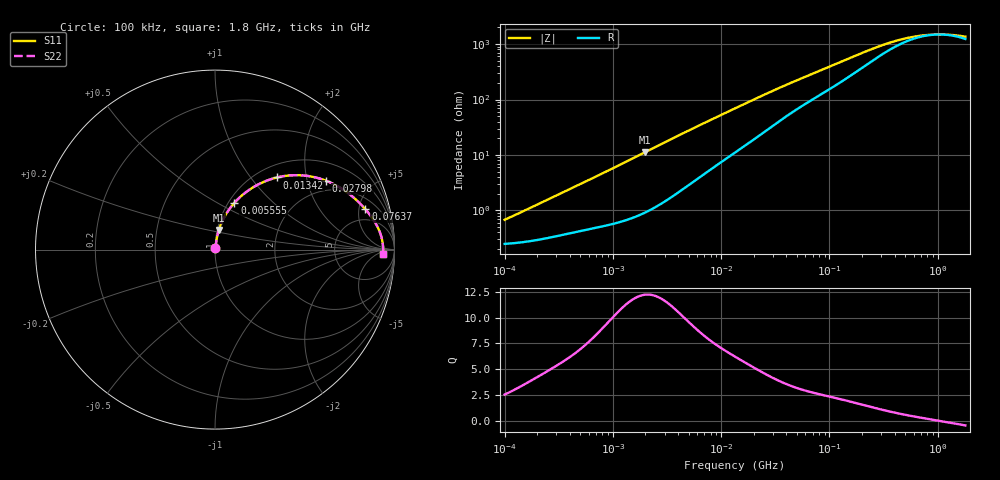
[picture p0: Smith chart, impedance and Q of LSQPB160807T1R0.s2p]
! LSQPB160807T1R0  S-PARAMETER MODEL  ( General Type )
! Model Generated by TAIYO YUDEN Corporation (http://www.ty-top.com)
! Version 1.0
! TAIYO YUDEN Control No. 110308NG25SB-FKC
! Copyright(c) 2011 TAIYO YUDEN CO.,LTD. All Rights Reserved.
! Product Description (link to TY-COMPAS)
! https://ds.yuden.co.jp/TYCOMPAS/or/detail?pn=LSQPB160807T1R0M&u=M
! Products Name : Inductors
! Characteristics :
!  Inductance : 1.0 uH , SRF(min) : 700 MHz , DC Resistance(max) : 0.299 Ohm
!  Rated Current : Saturation :510 mA , Temp Rise : 650 mA (40 degC)
!  Case Size : 1.6 x 0.8 / 0.063 x 0.031 [mm/inch] , Thickness : 0.7 / 0.028 [mm/inch]
!  (Conditions: Temperature = 25 degC , DC Bias Current/Voltage = 0A / 0V)
! External Node Assignments :
!  1  o---GGG---o  2
! GND o---------o GND
! Frequency Range : 0.1MHz  -  1800MHz  [ 402 STEP ]
# MHz S RI R 50
! Freq[MHz].  S11 Real  S11 Imag  S21 Real  S21 Imag  S12 Real  S12 Imag  S22 Real  S22 Imag
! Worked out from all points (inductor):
!   401 points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, 100 kHz to 1.8 GHz, reference 50 ohm
!   read as one part in series: L = 994 nH near 124.7 kHz
!   highest Q = 12.2 at 1.985 MHz (marker M1), where L = 898 nH
!   self-resonance near 1.02 GHz
!   S11 on the Smith chart (normalised r, x): 100 kHz: 1.00, +0.01; 5.555 MHz: 1.07, +0.60; 13.42 MHz: 1.22, +1.37; 27.98 MHz: 1.61, +2.63; 76.37 MHz: 3.23, +5.86; 1.8 GHz: 26, -11
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0.1  0.00252 0.00627  0.9975 -0.00627  0.9975 -0.00627  0.00252 0.00627
0.137498  0.0027 0.00856  0.9973 -0.00856  0.9973 -0.00856  0.0027 0.00856
0.516129  0.00519 0.0301  0.9948 -0.0301  0.9948 -0.0301  0.00519 0.0301
1.076226  0.00958 0.0606  0.9904 -0.0606  0.9904 -0.0606  0.00958 0.0606
1.985446  0.0211 0.1086  0.9789 -0.1086  0.9789 -0.1086  0.0211 0.1086
2.66389  0.0333 0.1425  0.9667 -0.1425  0.9667 -0.1425  0.0333 0.1425
3.942096  0.063 0.2004  0.937 -0.2004  0.937 -0.2004  0.063 0.2004
5.554714  0.1084 0.261  0.8916 -0.261  0.8916 -0.261  0.1084 0.261
8.632747  0.2044 0.3421  0.7956 -0.3421  0.7956 -0.3421  0.2044 0.3421
13.41641  0.3467 0.4023  0.6533 -0.4023  0.6533 -0.4023  0.3467 0.4023
19.37354  0.4872 0.4135  0.5128 -0.4135  0.5128 -0.4135  0.4872 0.4135
27.97575  0.6201 0.3832  0.3799 -0.3832  0.3799 -0.3832  0.6201 0.3832
42.42587  0.7358 0.3192  0.2642 -0.3192  0.2642 -0.3192  0.7358 0.3192
69.24595  0.8249 0.2393  0.1751 -0.2393  0.1751 -0.2393  0.8249 0.2393
76.37428  0.8382 0.2244  0.1618 -0.2244  0.1618 -0.2244  0.8382 0.2244
151.6408  0.9021 0.1333  0.0979 -0.1333  0.0979 -0.1333  0.9021 0.1333
253.6402  0.9238 0.0815  0.0762 -0.0815  0.0762 -0.0815  0.9238 0.0815
357.3983  0.9308 0.0552  0.0692 -0.0552  0.0692 -0.0552  0.9308 0.0552
542.0029  0.935 0.0302  0.065 -0.0302  0.065 -0.0302  0.935 0.0302
802.0705  0.9367 0.0109  0.0633 -0.0109  0.0633 -0.0109  0.9367 0.0109
1186.925  0.9371 -0.00683  0.0629 0.00683  0.0629 0.00683  0.9371 -0.00683
1800  0.9366 -0.0269  0.0634 0.0269  0.0634 0.0269  0.9366 -0.0269
